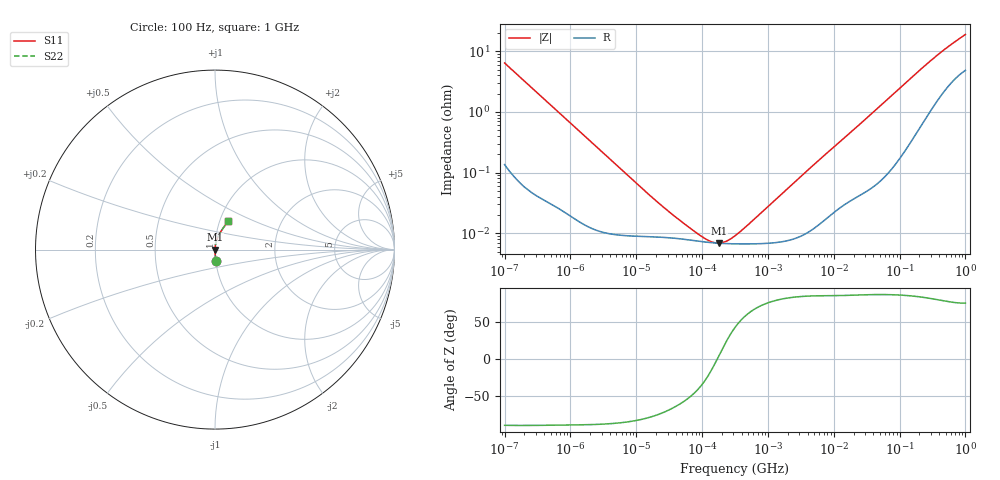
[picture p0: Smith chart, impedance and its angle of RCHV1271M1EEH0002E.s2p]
! RCHV1271M1EEH0002E  S-PARAMETER MODEL  (AEC-Q200 qualified)
! Model Generated by ELNA Corporation (http://www.ty-top.com)
! Version 1.0
! ELNA Control No. 240229
! Copyright (c) 2024 ELNA CO.,LTD. All Rights Reserved.
! Products Name : CONDUCTIVE POLYMER HYBRID ALUMINUM ELECTROLYTIC CAPACITORS
! Characteristics :
!  Capacitance  :  270uF  ,  Rated voltage  :  16V
!  Operating Temp. Range  :  -55 to +105 degC  ,  Endurance  :  10000hr at 105 degC
!  Dimension D  :  8mm  ,  Dimension L  :  10mm
! Frequency Range : 100Hz - 1GHz
! External Node Assignments :
!  1  o---| |---o  2
# MHz S RI R 50
!Freq[MHz].  S11 Real  S11 Imag  S21 Real  S21 Imag  S12 Real  S12 Imag  S22 Real  S22 Imag
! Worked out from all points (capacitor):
!   401 points, 100 Hz to 1 GHz, reference 50 ohm
!   read as one part in series: C = 248 uF near 108 Hz
!   lowest |Z| = 6.87 mohm at 179.9 kHz (marker M1)
!   series resonance near 169.7 kHz, so ESL is about 3.5 nH
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0.0001  0.00543 -0.0637  0.9946 0.0637  0.9946 0.0637  0.00543 -0.0637
0.000113  0.00434 -0.0565  0.9957 0.0565  0.9957 0.0565  0.00434 -0.0565
0.000309  0.000844 -0.0208  0.9992 0.0208  0.9992 0.0208  0.000844 -0.0208
0.001488  0.000165 -0.00441  0.9998 0.00441  0.9998 0.00441  0.000165 -0.00441
0.009495  9e-05 -0.000696  0.9999 0.000696  0.9999 0.000696  9e-05 -0.000696
0.022131  8.64e-05 -0.000299  0.9999 0.000299  0.9999 0.000299  8.64e-05 -0.000299
0.04217  8.19e-05 -0.000155  0.9999 0.000155  0.9999 0.000155  8.19e-05 -0.000155
0.080353  7.49e-05 -7.12e-05  0.9999 7.12e-05  0.9999 7.12e-05  7.49e-05 -7.12e-05
0.090678  7.36e-05 -5.87e-05  0.9999 5.87e-05  0.9999 5.87e-05  7.36e-05 -5.87e-05
0.179887  6.85e-05 5.32e-06  0.9999 -5.32e-06  0.9999 -5.32e-06  6.85e-05 5.32e-06
0.316228  6.69e-05 6.13e-05  0.9999 -6.13e-05  0.9999 -6.13e-05  6.69e-05 6.13e-05
0.356862  6.68e-05 7.54e-05  0.9999 -7.54e-05  0.9999 -7.54e-05  6.68e-05 7.54e-05
0.386812  6.67e-05 8.53e-05  0.9999 -8.53e-05  0.9999 -8.53e-05  6.67e-05 8.53e-05
0.419276  6.67e-05 9.58e-05  0.9999 -9.58e-05  0.9999 -9.58e-05  6.67e-05 9.58e-05
4.704354  0.000116 0.00127  0.9999 -0.00127  0.9999 -0.00127  0.000116 0.00127
25.55642  0.000468 0.00641  0.9995 -0.00641  0.9995 -0.00641  0.000468 0.00641
69.9842  0.00132 0.0172  0.9987 -0.0172  0.9987 -0.0172  0.00132 0.0172
163.1173  0.00527 0.0391  0.9947 -0.0391  0.9947 -0.0391  0.00527 0.0391
336.8992  0.0184 0.075  0.9816 -0.075  0.9816 -0.075  0.0184 0.075
592.2431  0.042 0.1149  0.958 -0.1149  0.958 -0.1149  0.042 0.1149
922.5714  0.0688 0.1533  0.9312 -0.1533  0.9312 -0.1533  0.0688 0.1533
1000  0.0743 0.1614  0.9257 -0.1614  0.9257 -0.1614  0.0743 0.1614
